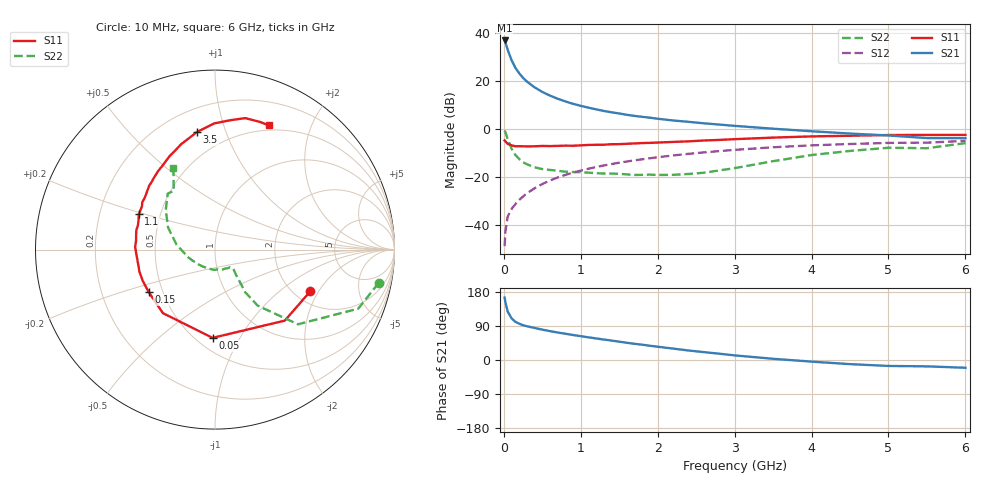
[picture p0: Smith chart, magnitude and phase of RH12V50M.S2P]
! SIEMENS Small Signal Semiconductors
! BFR106
! Si NPN RF Bipolar Junction Transistor in SOT23
! VCE = 12 V  IC = 50 mA
! Common Emitter S-Parameters:  August  1996
# GHz  S  MA  R  50
!  f  S11  S21  S12  S22
! GHz  MAG  ANG  MAG  ANG  MAG  ANG  MAG  ANG
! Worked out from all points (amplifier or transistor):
!   36 points, 10 MHz to 6 GHz, reference 50 ohm
!   highest |S21| = 36.8 dB at 10 MHz (marker M1)
!   |S21| within 3 dB of that: start of sweep to 41.91 MHz
!   unconditionally stable (mu >= 1): 270.4 MHz to 2.344 GHz
!   at 250 MHz: K = 0.99, MSG = 24.6 dB, |S12| = -28.0 dB
!   at 1.4 GHz: K = 1.07, MAG = 9.2 dB, |S12| = -14.5 dB
!   at 6 GHz: K = 0.97, MSG = 0.6 dB, |S12| = -4.9 dB
!   S11 on the Smith chart (normalised r, x): 10 MHz: 2.43, -1.70; 50 MHz: 0.60, -0.77; 150 MHz: 0.42, -0.24; 1.1 GHz: 0.38, +0.19; 3.5 GHz: 0.34, +0.80; 6 GHz: 0.44, +1.43
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0.01  0.5798 -23.6  69 164.7  0.0037 81.3  0.9308 -11.5
0.02  0.5548 -45.5  63.61 152.8  0.0074 74.7  0.8634 -22.4
0.05  0.492 -91.6  44.31 128.0  0.0152 61.0  0.622 -42.0
0.1  0.4578 -129.4  26.89 110.0  0.0219 59.9  0.3927 -52.7
0.15  0.4386 -147.6  18.7 100.9  0.0276 61.8  0.2896 -54.7
0.2  0.4386 -156.8  14.34 95.8  0.0338 64.5  0.239 -52.9
0.25  0.4386 -163.7  11.53 91.8  0.0397 66.4  0.2037 -51.4
0.3  0.436 -168.3  9.673 89.1  0.0464 68.0  0.1859 -50.5
0.4  0.4384 -176.2  7.333 84.5  0.059 69.6  0.1603 -47.9
0.5  0.4455 178.1  5.889 80.1  0.0722 70.3  0.1475 -46.2
0.6  0.4425 173.8  4.939 76.2  0.0855 70.0  0.1416 -46.6
0.7  0.4468 169.6  4.255 72.5  0.0984 69.8  0.1363 -48.3
0.9  0.4499 162.7  3.336 66.0  0.1248 68.2  0.1279 -50.4
1.1  0.4679 155.1  2.776 59.8  0.1498 66.1  0.1242 -57.3
1.3  0.4723 149.6  2.374 54.0  0.1753 63.7  0.1192 -63.6
1.6  0.4937 140.8  1.973 45.4  0.2118 60.0  0.1143 -77.1
2.2  0.5401 125.9  1.506 30.1  0.2831 52.1  0.112 -111.2
3  0.6159 108.0  1.164 12.2  0.3694 41.0  0.1543 -163.4
3.5  0.6635 98.6  1.016 3.2  0.4181 33.8  0.2151 173.0
4.5  0.7251 83.5  0.806 -10.9  0.4888 19.3  0.3512 141.4
5.5  0.7543 70.6  0.649 -16.8  0.5216 8.8  0.3997 125.1
6  0.7544 66.7  0.645 -20.5  0.5678 1.8  0.5097 117.0
